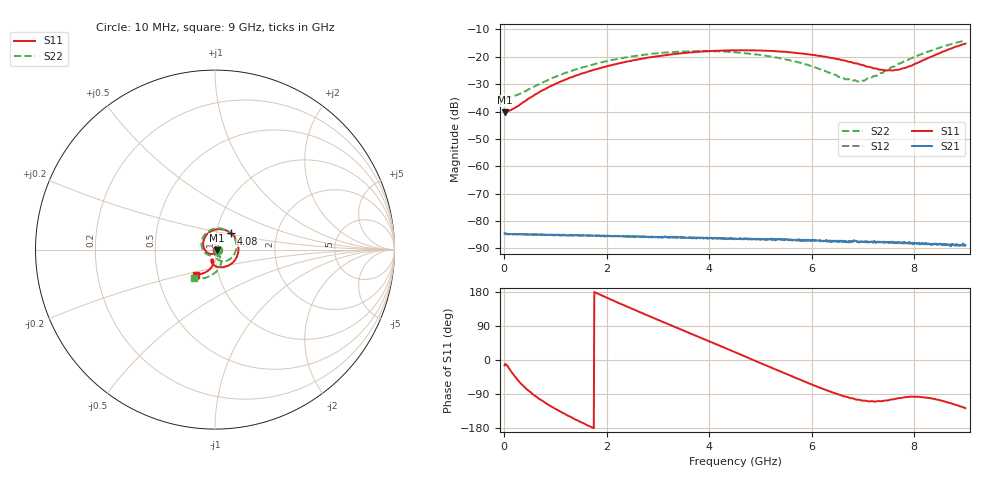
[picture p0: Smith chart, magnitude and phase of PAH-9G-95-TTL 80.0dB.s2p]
! MTS Systemtechnik GmbH
! S-Parameters
! Model: PAH-9G/95-TTL
! Attenuation Step: 80.0dB
#  HZ  S  DB  R  50.00
! Rohde & Schwarz Vector Network Analyzer
! Rohde-Schwarz,ZNB20-2Port,1334333062101652,3.45
! Created: UTC 1/26/2024, 7:24:43 AM
! freq[Hz]  db:S11  ang:S11  db:S21  ang:S21  db:S12  ang:S12  db:S22  ang:S22
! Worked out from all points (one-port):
!   900 points, 10 MHz to 9 GHz, reference 50 ohm
!   lowest |S11| = -40.2 dB at 20 MHz (marker M1), VSWR 1.02, Z = 51 - j0.186 ohm
!   |S11| at or under -10 dB: start of sweep to end of sweep
!   S11 on the Smith chart (normalised r, x): 10 MHz: 1.02, -0.00; 4.08 GHz: 1.18, +0.22; 9 GHz: 0.78, -0.22
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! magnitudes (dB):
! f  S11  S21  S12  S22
! 10 MHz  -40.1  -84.6  -84.7  -35.2
! 20 MHz  -40.2  -84.6  -84.7  -35.2
! 140 MHz  -39.4  -84.7  -84.7  -34.8
! 290 MHz  -37.8  -84.9  -84.9  -33.7
! 600 MHz  -33.9  -85.0  -85.0  -30.8
! 890 MHz  -30.9  -84.9  -85.1  -28.2
! 1.51 GHz  -26.1  -85.3  -85.4  -24.0
! 2.14 GHz  -22.8  -85.5  -85.5  -21.0
! 3.01 GHz  -19.8  -85.7  -86.1  -18.7
! 4.08 GHz  -17.9  -86.3  -86.2  -18.0
! 4.51 GHz  -17.7  -86.3  -86.6  -18.4
! 5.31 GHz  -18.0  -86.6  -86.6  -20.2
! 6.01 GHz  -19.3  -86.9  -87.2  -23.5
! 6.66 GHz  -21.5  -87.6  -87.6  -28.2
! 6.9 GHz  -22.5  -87.4  -87.6  -29.0
! 7.14 GHz  -23.8  -87.8  -87.7  -28.0
! 7.33 GHz  -24.7  -87.5  -87.8  -26.0
! 7.51 GHz  -24.9  -87.8  -87.8  -24.5
! 7.69 GHz  -24.8  -88.0  -88.2  -22.7
! 7.84 GHz  -24.0  -88.0  -88.1  -21.4
! 8.48 GHz  -18.8  -88.6  -88.4  -16.7
! 9 GHz  -15.2  -88.8  -88.9  -14.0
